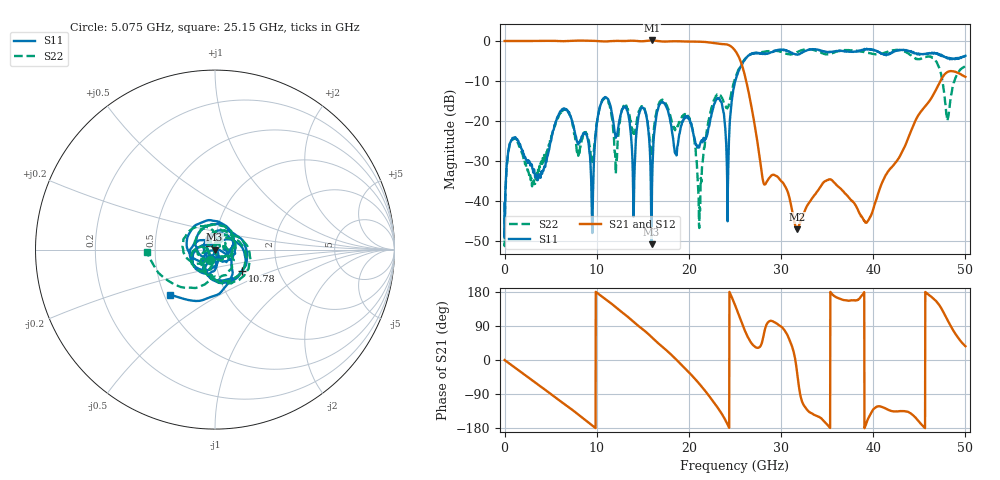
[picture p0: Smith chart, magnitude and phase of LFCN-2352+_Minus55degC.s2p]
! Mini-Circuits
! S2P DATA File Format
! Type: LOW PASS FILTER
! Model: LFCN-2352+
! All S Parameters are in dB deg format
! TEST CONDITIONS: INPUT POWER = 0 dBm - -55 deg C
# MHZ S DB R 50
!Frequency  S11 dB  S11 DEG  S21 dB  S21 DEG  S12 dB  S12 DEG  S22 dB  S22 DEG
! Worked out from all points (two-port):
!   2006 points, 10 MHz to 50 GHz, reference 50 ohm
!   highest |S21| = 0.13 dB at 16 GHz (marker M1); lowest = -47.0 dB at 31.75 GHz (marker M2)
!   |S21| within 3 dB of the highest: start of sweep to 25.16 GHz
!   lowest |S11| = -50.8 dB at 15.95 GHz (marker M3), VSWR 1.01, Z = 49.7 - j0.127 ohm
!   |S11| at or under -10 dB: start of sweep to 25.04 GHz
!   |S22| runs from -51.3 to -2.1 dB; largest |S21 - S12| = 0.0038
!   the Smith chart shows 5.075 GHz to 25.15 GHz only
!   S11 on the Smith chart (normalised r, x): 5.075 GHz: 0.94, -0.10; 10.78 GHz: 1.31, -0.33; 25.15 GHz: 0.54, -0.31
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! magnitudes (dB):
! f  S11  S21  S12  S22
! 10 MHz  -40.5  0.0  0.0  -40.4
! 800 MHz  -24.8  0.0  0.0  -24.8
! 5.075 GHz  -24.5  0.0  0.0  -23.7
! 8.35 GHz  -24.0  0.1  0.1  -25.0
! 9.525 GHz  -48.0  0.0  0.0  -30.2
! 10.78 GHz  -14.2  -0.1  -0.1  -14.3
! 15.1 GHz  -16.9  -0.1  -0.1  -16.8
! 15.95 GHz  -50.8  0.1  0.1  -28.5
! 16 GHz  -36.7  0.1  0.1  -27.5
! 16.68 GHz  -16.8  0.0  0.0  -16.1
! 20 GHz  -19.3  -0.2  -0.2  -19.4
! 21.15 GHz  -26.2  -0.2  -0.2  -43.0
! 23.23 GHz  -14.3  -0.7  -0.7  -13.3
! 24.2 GHz  -45.0  -0.9  -0.9  -16.7
! 25.02 GHz  -10.1  -2.4  -2.4  -9.2
! 25.15 GHz  -9.0  -2.8  -2.8  -8.4
! 28.1 GHz  -3.1  -35.5  -35.5  -2.7
! 31.75 GHz  -3.4  -47.0  -47.0  -2.7
! 33.35 GHz  -2.1  -39.4  -39.4  -2.2
! 41.67 GHz  -3.3  -32.4  -32.4  -2.6
! 48.08 GHz  -4.4  -7.7  -7.7  -19.6
! 50 GHz  -3.7  -9.0  -9.0  -6.2
